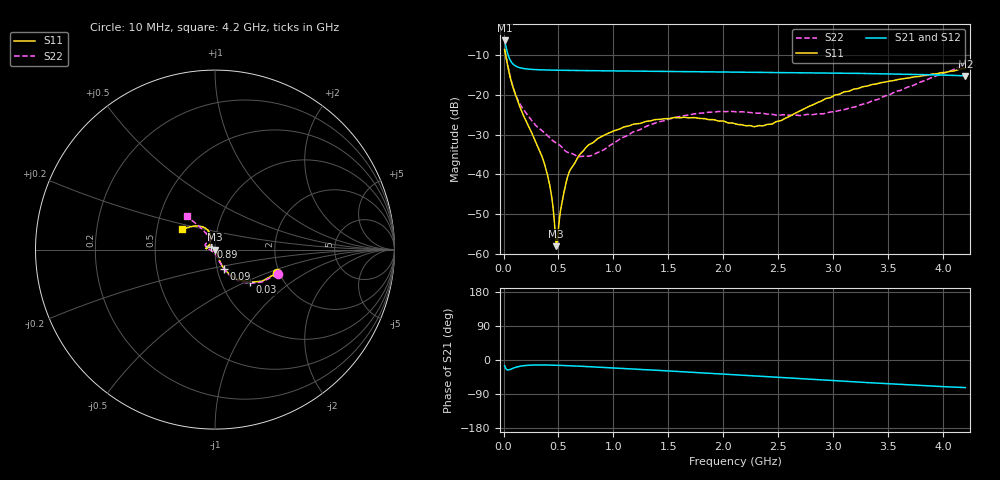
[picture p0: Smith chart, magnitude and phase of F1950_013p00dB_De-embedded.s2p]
! Integrated Device Technology
! Corporate Headquarters
! 6024 Silver Creek Valley Road
! San Jose, CA 95138  USA
! Phone:  1-408-284-8200
! Toll Free:  1-800-223-1366
! Webpage:  http://www.idt.com/
! Timing and RF Division
! 515 Groton Road, Suite 102
! Westford, MA 01886-6024
! Device:  F1950
! Description: 7-bit 0.25 dB Digital Step Attenuator
! Frequency:  150.0 -  4000.00 MHz
! Package:  4x4 mm Thin QFN Plastic Package: 24 pin
! Ports:  2 RF, 12 DC
!  Pin  1  = D0
!  Pin  2  = VDD
!  Pin  3  = Vmode
!  Pin  4  = GND
!  Pin  5  = RF1  =  Port 1
!  Pin  6  = GND
!  Pin  7  = GND
!  Pin  8  = GND
!  Pin  9  = GND
!  Pin 10  = GND
!  Pin 11  = GND
!  Pin 12  = GND
!  Pin 13  = GND
!  Pin 14  = RF2  =  Port 2
!  Pin 15  = GND
!  Pin 16  = LE
!  Pin 17  = CLK
!  Pin 18  = DATE
!  Pin 19  = D6
!  Pin 20  = D5
!  Pin 21  = D4
!  Pin 22  = D3
!  Pin 23  = D2
!  Pin 24  = D1
! State:  52
! Atten State:  13.00 dB
! Voltage:  +5.00 Volts
! Current:  Not Measured mA
! Data:  The device was measured on a the F195X evaluation board which has
!  individual transmission lines to the RF pins.  Data was collected
!  using a calibrated network analyzer.  The evaluation board was
!  de-embedded using a TRL calibration technique.
!  The reference plane is the edge of the package pin.
! Misc:  Board 2019
!  Action Tracker AT0250
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# GHz S dB R 50
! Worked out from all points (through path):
!   420 points, 10 MHz to 4.2 GHz, reference 50 ohm
!   highest |S21| = -6.35 dB at 10 MHz (marker M1); lowest = -15.2 dB at 4.2 GHz (marker M2)
!   group delay of S21, straight-line fit = 42.7 ps
!   lowest |S11| = -58.0 dB at 480 MHz (marker M3), VSWR 1.00, Z = 50.1 + j0.0514 ohm
!   |S11| at or under -10 dB: 19.83 MHz to end of sweep
!   |S22| runs from -35.5 to -8.5 dB; largest |S21 - S12| = 0.00029
!   S11 on the Smith chart (normalised r, x): 10 MHz: 1.95, -0.58; 30 MHz: 1.36, -0.53; 90 MHz: 1.08, -0.24; 890 MHz: 0.95, +0.03; 4.2 GHz: 0.67, +0.16
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0.01  -8.61 -20.3  -6.35 -15.1  -6.35 -15.1  -8.52 -21.1
0.03  -11.52 -43.3  -8.80 -25.4  -8.79 -25.4  -11.43 -44.6
0.06  -15.55 -58.2  -11.25 -25.0  -11.25 -25.0  -15.30 -59.5
0.09  -18.46 -64.4  -12.38 -21.4  -12.38 -21.4  -18.37 -64.5
0.18  -25.12 -65.8  -13.39 -15.1  -13.39 -15.1  -23.64 -71.1
0.38  -38.10 -53.8  -13.77 -13.2  -13.77 -13.2  -29.74 -77.8
0.43  -44.23 -48.6  -13.80 -13.5  -13.80 -13.5  -31.08 -80.5
0.47  -54.62 -13.5  -13.83 -13.8  -13.82 -13.8  -31.96 -85.9
0.48  -58.05 24.2  -13.83 -13.9  -13.83 -13.9  -32.12 -86.9
0.5  -53.44 96.7  -13.84 -14.0  -13.84 -14.1  -32.45 -88.4
0.54  -45.90 120.7  -13.86 -14.5  -13.86 -14.5  -33.49 -91.2
0.59  -40.00 126.9  -13.88 -15.0  -13.88 -15.1  -34.49 -101.2
0.71  -34.54 135.3  -13.92 -16.6  -13.92 -16.6  -35.48 -122.9
0.89  -30.54 145.0  -13.97 -19.2  -13.97 -19.2  -34.11 -157.4
1.41  -26.20 167.7  -14.11 -27.4  -14.11 -27.4  -26.83 167.1
1.73  -25.73 174.3  -14.19 -32.7  -14.19 -32.7  -24.82 158.5
2.11  -27.34 165.6  -14.29 -39.1  -14.28 -39.2  -24.27 148.9
2.43  -27.44 132.9  -14.37 -44.5  -14.37 -44.5  -24.88 138.7
2.81  -22.57 108.6  -14.47 -51.1  -14.47 -51.1  -25.00 123.1
3.19  -18.55 111.2  -14.61 -57.6  -14.60 -57.7  -23.09 116.7
3.51  -16.56 120.0  -14.75 -62.9  -14.74 -62.9  -20.00 118.5
4.2  -13.28 148.0  -15.25 -72.7  -15.24 -72.8  -12.30 130.1
